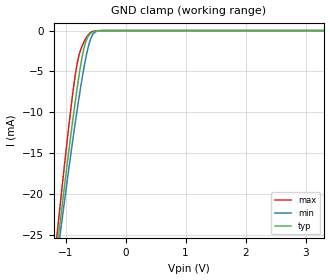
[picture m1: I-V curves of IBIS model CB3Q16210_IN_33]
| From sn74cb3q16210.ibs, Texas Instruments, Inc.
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[Model]   CB3Q16210_IN_33
Model_type  Input
Vinl=0.8
Vinh=2.0
| variable   typ   min   max
C_comp   2.82pF   2.06pF   3.42pF
[Temperature Range]   40   100   -40
| Ambient temperature   25   85   -40
[Voltage range]   3.3   3   3.6
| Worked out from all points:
|   GND clamp passes 1 mA (typ) near -0.64 V on its own axis
[GND Clamp]
| CB3Q16210_IN_33
|   Voltage   I(typ)   I(min)   I(max)
-5.5V     -337.1mA   -312.5mA   -365.5mA
-1.155V   -27.6mA    -28.73mA   -25.97mA
-1.115V   -25.08mA   -26.43mA   -23.16mA
-1.08V    -22.9mA    -24.44mA   -20.72mA
-895mV    -11.85mA   -14.26mA   -8.606mA
-835mV    -8.541mA   -11.15mA   -5.317mA
-795mV    -6.475mA   -9.162mA   -3.631mA
-720mV    -3.119mA   -5.681mA   -1.83mA
-665mV    -1.423mA   -3.455mA   -1.004mA
-585mV    -361.7uA   -1.1mA     -263.4uA
-510mV    -78.74uA   -202.2uA   -38.8uA
3.3V      76.2pA     212.5pA    43.07pA
